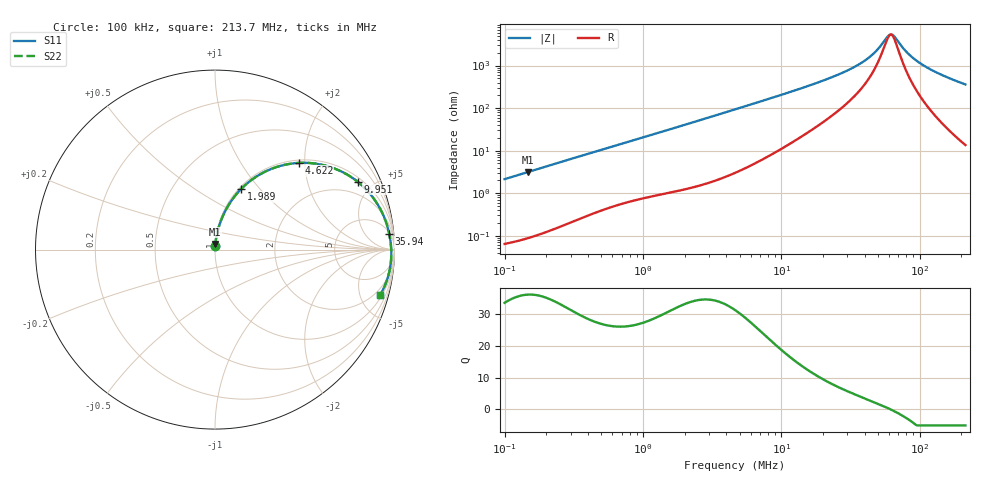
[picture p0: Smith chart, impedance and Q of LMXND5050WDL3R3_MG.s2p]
! LMXND5050WDL3R3_MG  S-PARAMETER MODEL  ( General Type )
! Model Generated by TAIYO YUDEN Corporation (https://www.yuden.co.jp/en/)
! Version 1.0
! TAIYO YUDEN Control No. 191023NI43SB-FBB
! Copyright(c) 2019 TAIYO YUDEN CO.,LTD. All Rights Reserved.
! Product Description (link to TY-COMPAS)
! https://ds.yuden.co.jp/TYCOMPAS/or/detail?pn=LMXND5050WDL3R3NMG&u=M
! Products Name : Inductors
! Characteristics :
!  Inductance : 3.3 uH , SRF(min) : 41 MHz , DC Resistance(max) : 0.0516 Ohm
!  Rated Current : Saturation :3100 mA , Temp Rise : 2400 mA (40 degC)
!  Case Size : 4.9 x 4.9 / 0.193 x 0.193 [mm/inch] , Thickness : 2.4 / 0.094 [mm/inch]
!  (Conditions: Temperature = 25 degC , DC Bias Current/Voltage = 0A / 0V)
! External Node Assignments :
!  1  o---GGG---o  2
! GND o---------o GND
! Frequency Range : 0.1MHz  -  213.673535MHz  [ 402 STEP ]
# MHz S RI R 50
! Freq[MHz].  S11 Real  S11 Imag  S21 Real  S21 Imag  S12 Real  S12 Imag  S22 Real  S22 Imag
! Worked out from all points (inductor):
!   401 points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, 100 kHz to 213.7 MHz, reference 50 ohm
!   read as one part in series: L = 3.39 uH near 103.9 kHz
!   highest Q = 35.9 at 146.7 kHz (marker M1), where L = 3.39 uH
!   self-resonance near 61.73 MHz
!   S11 on the Smith chart (normalised r, x): 100 kHz: 1.00, +0.04; 1.989 MHz: 1.02, +0.80; 4.622 MHz: 1.06, +1.86; 9.951 MHz: 1.22, +4.08; 35.94 MHz: 6, +20; 213.7 MHz: 1.27, -7.20
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0.1  0.00109 0.0213  0.9989 -0.0213  0.9989 -0.0213  0.00109 0.0213
0.146719  0.00184 0.0312  0.9982 -0.0312  0.9982 -0.0312  0.00184 0.0312
0.361188  0.0083 0.0752  0.9917 -0.0752  0.9917 -0.0752  0.0083 0.0752
0.72013  0.0269 0.1438  0.9731 -0.1438  0.9731 -0.1438  0.0269 0.1438
1.304567  0.0729 0.2433  0.9271 -0.2433  0.9271 -0.2433  0.0729 0.2433
1.988853  0.1462 0.3385  0.8538 -0.3385  0.8538 -0.3385  0.1462 0.3385
2.974505  0.2699 0.4296  0.7301 -0.4296  0.7301 -0.4296  0.2699 0.4296
4.622483  0.4659 0.483  0.5341 -0.483  0.5341 -0.483  0.4659 0.483
4.71194  0.4752 0.4835  0.5248 -0.4835  0.5248 -0.4835  0.4752 0.4835
6.653322  0.6397 0.4609  0.3603 -0.4609  0.3603 -0.4609  0.6397 0.4609
9.950627  0.7941 0.3785  0.2059 -0.3785  0.2059 -0.3785  0.7941 0.3785
16.69585  0.9093 0.2469  0.0907 -0.2469  0.0907 -0.2469  0.9093 0.2469
25.94593  0.9543 0.149  0.0457 -0.149  0.0457 -0.149  0.9543 0.149
35.94047  0.9706 0.0885  0.0294 -0.0885  0.0294 -0.0885  0.9706 0.0885
46.11058  0.9777 0.0469  0.0223 -0.0469  0.0223 -0.0469  0.9777 0.0469
60.30341  0.9817 0.00374  0.0183 -0.00374  0.0183 -0.00374  0.9817 0.00374
62.66003  0.9819 -0.00243  0.0181 0.00243  0.0181 0.00243  0.9819 -0.00243
65.10875  0.9821 -0.00863  0.0179 0.00863  0.0179 0.00863  0.9821 -0.00863
81.94678  0.9817 -0.047  0.0183 0.047  0.0183 0.047  0.9817 -0.047
103.1394  0.9777 -0.0883  0.0223 0.0883  0.0223 0.0883  0.9777 -0.0883
142.8693  0.9629 -0.155  0.0371 0.155  0.0371 0.155  0.9629 -0.155
213.6735  0.9203 -0.2527  0.0797 0.2527  0.0797 0.2527  0.9203 -0.2527
